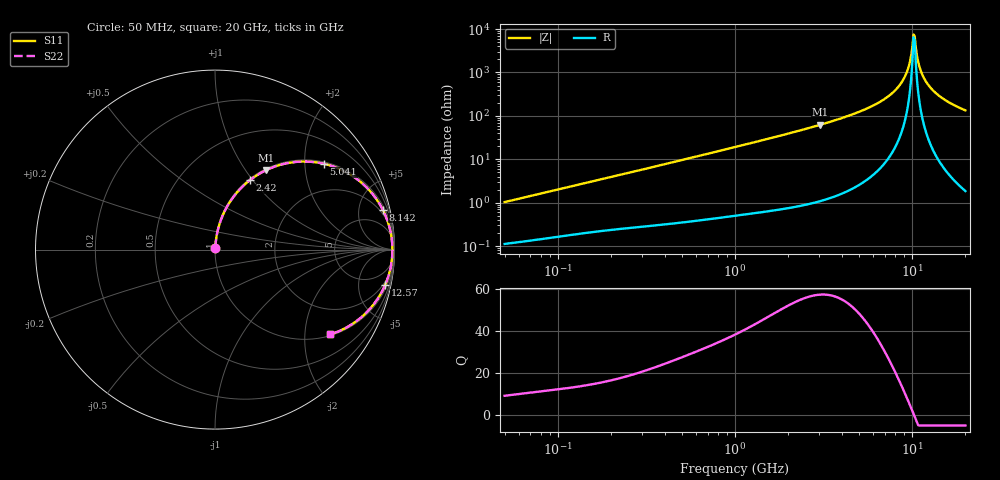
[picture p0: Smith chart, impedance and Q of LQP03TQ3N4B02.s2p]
!Murata Part Number: LQP03TQ3N4B02
!These Parameters are Measured in Series Mode Connection
!  o--[Z]--o
!Port1  Port2
!  o-------o
!Freq. Start=50[MHz] Stop=20[GHz], 401[Steps]
# Hz S RI R 50
!Freq.(Hz) S11(Real) S11(Imag) S21(Real) S21(Imag) S12(Real) S12(Imag) S22(Real) S22(Imag)
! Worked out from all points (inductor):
!   401 points, 50 MHz to 20 GHz, reference 50 ohm
!   read as one part in series: L = 3.25 nH near 51.52 MHz
!   highest Q = 57.3 at 3.03 GHz (marker M1), where L = 3.28 nH
!   self-resonance near 10.19 GHz
!   S11 on the Smith chart (normalised r, x): 50 MHz: 1.00, +0.02; 2.42 GHz: 1.02, +0.97; 5.041 GHz: 1.05, +2.50; 8.142 GHz: 1.43, +8.25; 12.57 GHz: 1.49, -9.39; 20 GHz: 1.04, -2.68
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5e7  0.00123 0.0103  0.9988 -0.0103  0.9988 -0.0103  0.00123 0.0103
1.364002e8  0.00269 0.0269  0.9973 -0.0269  0.9973 -0.0269  0.00269 0.0269
3.721004e8  0.00814 0.071  0.9919 -0.071  0.9919 -0.071  0.00814 0.071
1e9  0.0399 0.1831  0.9601 -0.1831  0.9601 -0.1831  0.0399 0.1831
2.419936e9  0.1933 0.386  0.8067 -0.386  0.8067 -0.386  0.1933 0.386
2.728004e9  0.2379 0.4171  0.7621 -0.4171  0.7621 -0.4171  0.2379 0.4171
3.029571e9  0.2841 0.4423  0.7159 -0.4423  0.7159 -0.4423  0.2841 0.4423
5.041459e9  0.6074 0.4781  0.3926 -0.4781  0.3926 -0.4781  0.6074 0.4781
6.311513e9  0.7784 0.402  0.2216 -0.402  0.2216 -0.402  0.7784 0.402
7.442007e9  0.8879 0.2968  0.1121 -0.2968  0.1121 -0.2968  0.8879 0.2968
8.141811e9  0.9343 0.2232  0.0657 -0.2232  0.0657 -0.2232  0.9343 0.2232
8.774992e9  0.9631 0.1548  0.0369 -0.1548  0.0369 -0.1548  0.9631 0.1548
9.316812e9  0.9787 0.0967  0.0213 -0.0967  0.0213 -0.0967  0.9787 0.0967
9.600142e9  0.9838 0.0669  0.0162 -0.0669  0.0162 -0.0669  0.9838 0.0669
1.004137e10  0.988 0.0216  0.012 -0.0216  0.012 -0.0216  0.988 0.0216
1.019291e10  0.9885 0.00646  0.0115 -0.00646  0.0115 -0.00646  0.9885 0.00646
1.050288e10  0.9881 -0.0239  0.0119 0.0239  0.0119 0.0239  0.9881 -0.0239
1.082228e10  0.9858 -0.0542  0.0142 0.0542  0.0142 0.0542  0.9858 -0.0542
1.131968e10  0.9788 -0.0991  0.0212 0.0991  0.0212 0.0991  0.9788 -0.0991
1.257102e10  0.9473 -0.199  0.0527 0.199  0.0527 0.199  0.9473 -0.199
1.527346e10  0.8414 -0.353  0.1586 0.353  0.1586 0.353  0.8414 -0.353
2e10  0.6409 -0.4729  0.3591 0.4729  0.3591 0.4729  0.6409 -0.4729
